FUNCTION_BLOCK FB12
TITLE =Get Encoder Parameter
//*****************************************************************************
//* maxon motor ag
//* R&D
//* all rights reserved
//*****************************************************************************
//* Summary:  Read encoder parameters
//*
//* Remarks:
//*
//* Created under: STEP7 REV5.2+SP1
//*****************************************************************************
//* History:
//* 19.05.2004 | INA   first release
//*
//*
//*****************************************************************************
//

AUTHOR:INA
FAMILY:Configur
NAME:GEncPara
VERSION:00.01


VAR_INPUT

Read : BOOL //A rising edge start the command

  NodeID : BYTE //Adress of the maxon device

END_VAR
VAR_OUTPUT
  Done : BOOL //Data valid flag is TRUE if data were available

  Err : BOOL //Error flag is TRUE if an Error has occured, see ErrNo for more details

  ErrNo : DINT //Contains detailed error information

  Counts : WORD //Incremental Encoder Counts

  PositionSensorType : WORD //Position Sensor Type

END_VAR
VAR
  xEdgeMerker : BOOL //Edge Merker

  xEdgeFlag : BOOL //Edge Flag

  xStep : INT
END_VAR

BEGIN

NETWORK
TITLE = Activate the service function
//

// SDO Read "Get Encoder Parameter"

       U    #Read
       FP   #xEdgeFlag                   // recognize a positiv edge of the Read signal
       =    #xEdgeMerker                 // and set the xEdgeMerker for one cycle to true

       L    #xStep
       L    0
       ==I
       U    #xEdgeMerker
       SPB  nstp                         // iStep = 1 -> fnc1

       L    #xStep                       // jump list
       SPL  List
       SPA  rdef
       SPA  fnc1
       SPA  fncE
List  :SPA  rdef

rdef  :NOP  0
       R    #Done                        // reset Done
       R    #Err                         // reset Error
       L    0
       T    #xStep                       // iStep = 0
       SPA  end

fnc1  :NOP  0
       CALL FC1
         NodeID:=#NodeID
         Index:=DW#16#00002210
         SubIndex:=DW#16#00000001        // Encoder Counts
         RET_VAL:=#Done
         Err:=#Err
         ErrNo:=#ErrNo

       L    DB219.DBW10
       T    #Counts

       L    1
       U    #Err
       SPB  fncE

       NOP  0
       CALL FC1
         NodeID:=#NodeID
         Index:=DW#16#00002210
         SubIndex:=DW#16#00000002        // Position Sensor Type
         RET_VAL:=#Done
         Err:=#Err
         ErrNo:=#ErrNo

       L    DB219.DBW10
       T    #PositionSensorType

fncE  :NOP  0
       L    0
       T    #xStep
       SPA  end

nstp  :NOP  0
       L    #xStep
       INC            1
       T    #xStep

end   :NOP  0
END_FUNCTION_BLOCK
